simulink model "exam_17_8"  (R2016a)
settings: Solver=ode23tb  StartTime=0.0  StopTime=0.0004  RelTol=1e-3
libraries: powerlib x11

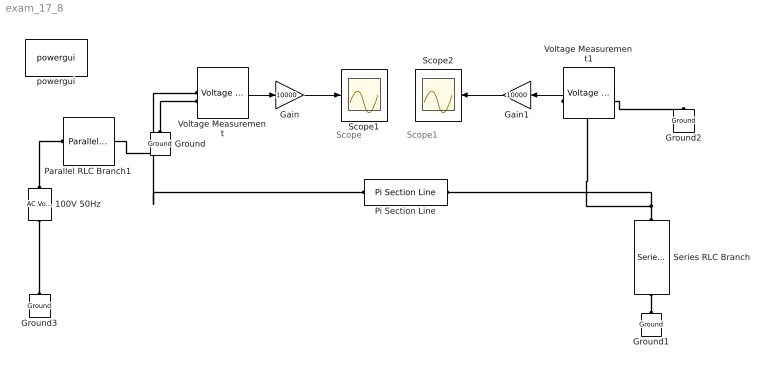
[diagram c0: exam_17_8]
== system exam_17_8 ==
  note: Scope1
  note: Scope
  100V 50Hz : powerlib/Electrical Sources/AC Voltage Source  Amplitude=100  Phase=0  Frequency=50  SampleTime=0  Measurements=None  BusType=swing  Pref=10e3  Qref=0  Qmin=-inf  Qmax=+inf
  Gain : Gain  Gain=10000
  Gain1 : Gain  Gain=10000
  Ground{,1..3} (4 alike) : powerlib/Elements/Ground  LConnTagsString=a
  Parallel RLC Branch1 : powerlib/Elements/Parallel RLC Branch  LConnTagsString=a  RConnTagsString=__new0  BranchType=R  Resistance=1  Inductance=1e-3  SetiL0=off  InitialCurrent=0  Capacitance=1e-6  Setx0=off  InitialVoltage=0  Measurements=None
  Pi Section Line : powerlib/Elements/Pi Section Line  LConnTagsString=__new0  RConnTagsString=__new0  Frequency=50  Resistance=0.1  Inductance=0.0016  Capacitance=0.0102e-6  Length=300  PiSections=10  Measurements=None
  Scope1 : Scope
  Scope2 : Scope
  Series RLC Branch : powerlib/Elements/Series RLC Branch  LConnTagsString=__new0  RConnTagsString=__new0  BranchType=RL  Resistance=1  Inductance=1  SetiL0=off  InitialCurrent=0  Capacitance=3.06e-6  Setx0=off  InitialVoltage=0  Measurements=None
  Voltage Measurement : powerlib/Measurements/Voltage Measurement  PhasorSimulation=off  OutputType=Complex  PSBequivalent=0
  Voltage Measurement1 : powerlib/Measurements/Voltage Measurement  PhasorSimulation=off  OutputType=Complex  PSBequivalent=0
  powergui : powerlib/powergui  Priority=1  SimulationMode=Discrete  SolverType=Tustin  SampleTime=25e-6  frequency=60  SPID=off  DisableSnubberDevices=off  DisableRonSwitches=off  DisableVfSwitches=off  SwTol=0  DisplayEquations=off  Interpol=off  ExternalGateDelay=off  methode=off  Ts=10  FunctionMessages=off  echomessages=off  HookPort=off  EnableUseOfTLC=off  x0status=blocks  frequencyindice=50  Pbase=100e6  ErrMax=1e-4  Iterations=50  UnitsV=kV  UnitsW=MW  buscounter=0  RestoreLinks=warning  ResistiveCurrentMeasurement=off  Frange=[0:2:500]  Ylog=on  Xlog=off  ShowGrid=on  save=off  variable=ZData  structure=0  ZoomFFT=off  StartTime=0.0  cycles=1  DisplayStyle=1  fundamental=60  FreqAxis=off  MaxFrequency=1000  frequencyindicesteady=1  RmsSteady=1  display=off
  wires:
  Voltage Measurement/1 -> Gain/1
  Gain/1 -> Scope1/1
  Gain1/1 -> Scope2/1
  Voltage Measurement1/1 -> Gain1/1
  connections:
  Voltage Measurement/LConn1 -- Parallel RLC Branch1/RConn1 -- Pi Section Line/LConn1
  Series RLC Branch/LConn1 -- Voltage Measurement1/LConn1 -- Pi Section Line/RConn1
  Ground/LConn1 -- Voltage Measurement/LConn2
  Series RLC Branch/RConn1 -- Ground1/LConn1
  Ground3/LConn1 -- 100V 50Hz/LConn1
  100V 50Hz/RConn1 -- Parallel RLC Branch1/LConn1
  Voltage Measurement1/LConn2 -- Ground2/LConn1
